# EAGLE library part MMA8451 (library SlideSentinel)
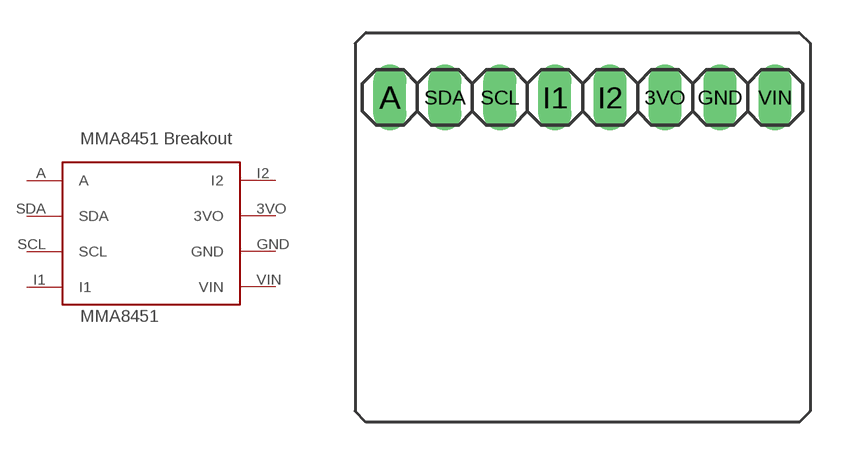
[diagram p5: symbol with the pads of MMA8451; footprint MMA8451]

Designator prefix -

## MMA8451  [MMA8451]
3VO  3VO
A  A
GND  GND
I1  I1
I2  I2
SCL  SCL
SDA  SDA
VIN  VIN

## Footprint MMA8451 (pad centres in mm)
PIN HEADER
drill 1.016 long: 3VO 3.81,0; A -8.89,0; GND 6.35,0; I1 -1.27,0; I2 1.27,0; SCL -3.81,0; SDA -6.35,0; VIN 8.89,0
